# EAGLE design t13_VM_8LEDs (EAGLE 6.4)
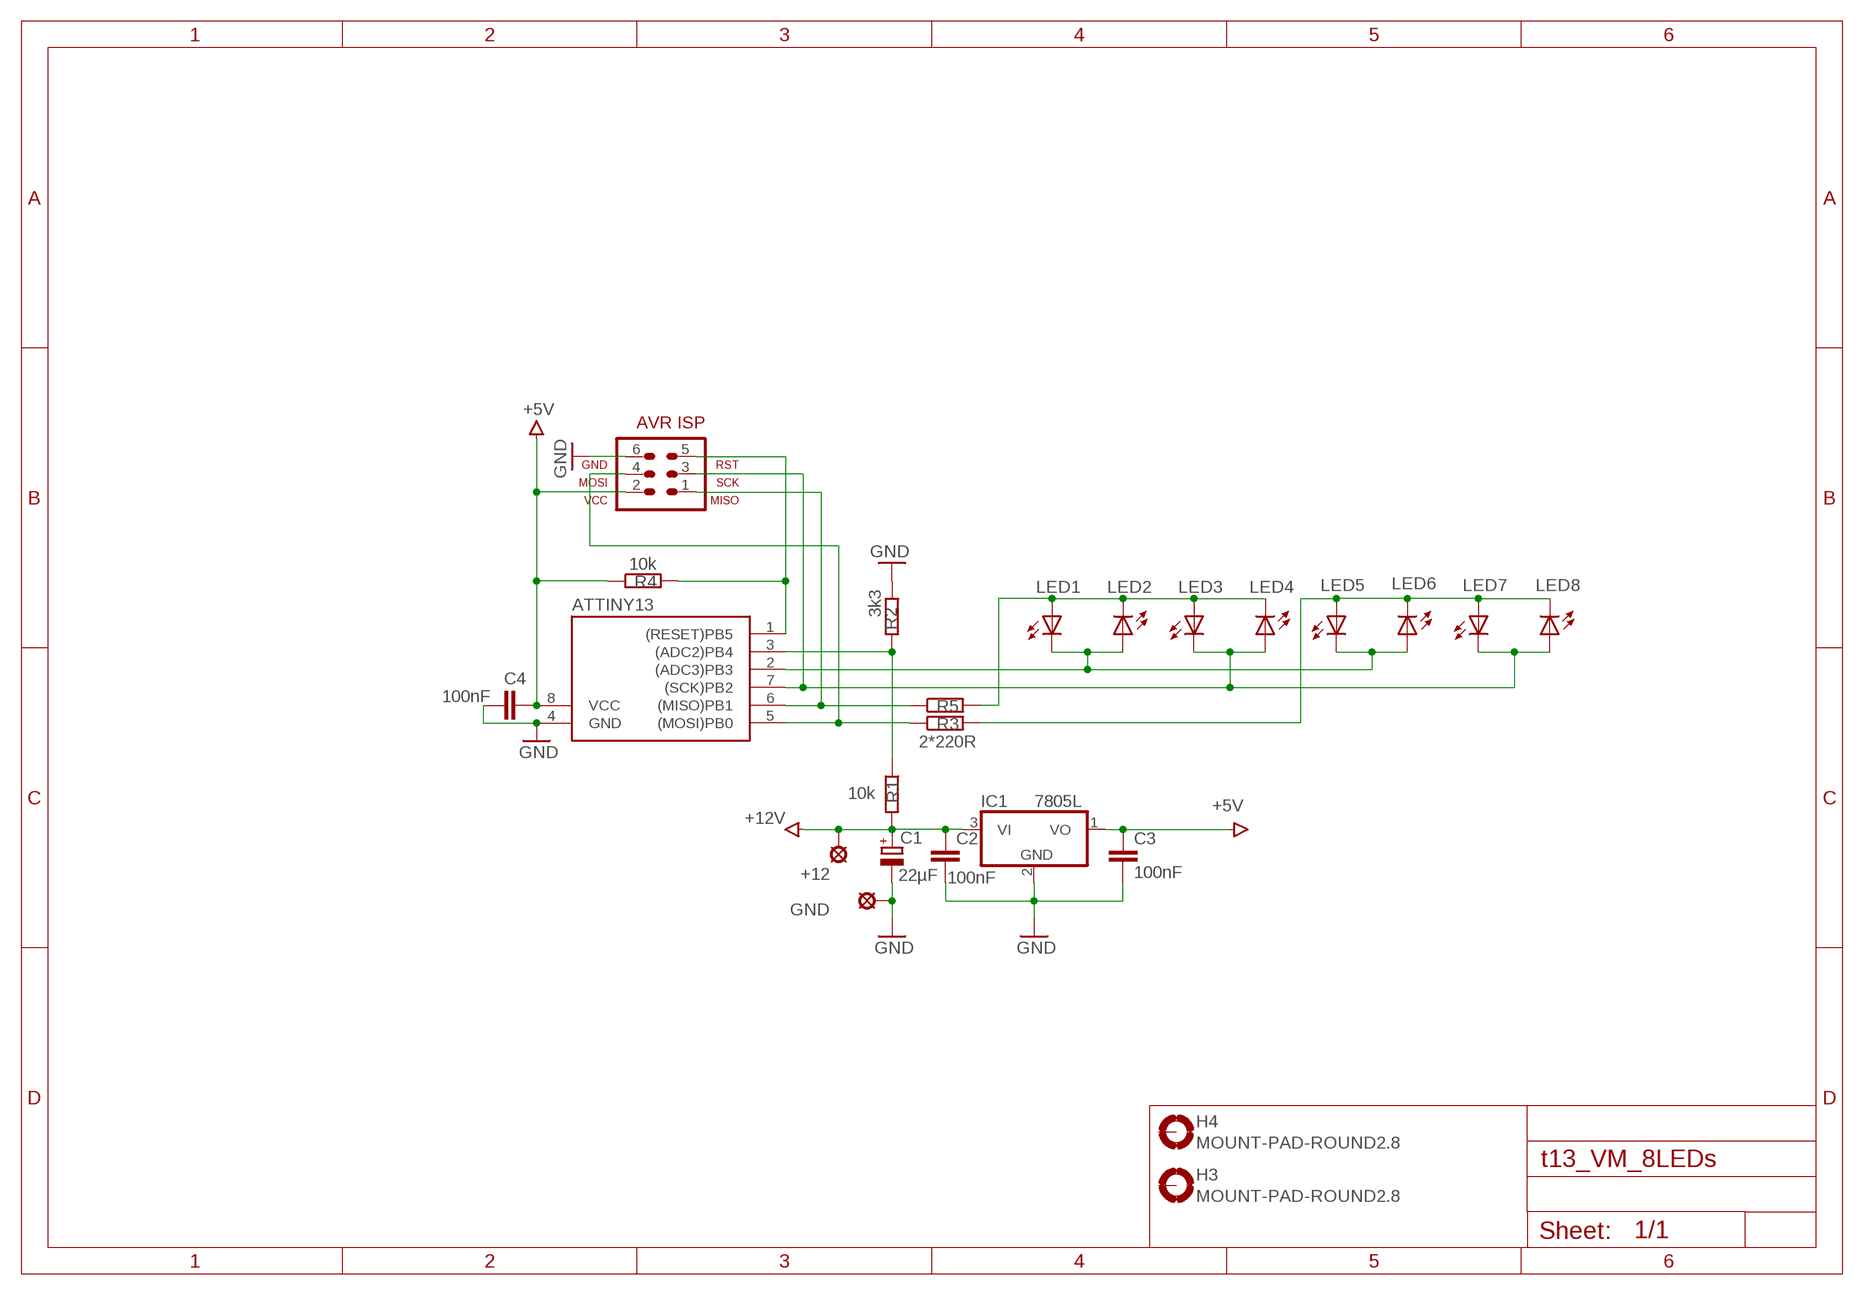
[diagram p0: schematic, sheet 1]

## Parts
+12  LSP10  [LSP10]
ATTINY13  TINY138P3  [DIL08]
C1  22µF  CPOL-EUE2.5-7  [E2,5-7]
C2  100nF  C-EU025-025X050  [C025-025X050]
C3  100nF  C-EU025-025X050  [C025-025X050]
C4  100nF  C-EU025-025X050  [C025-025X050]
GND  GND  LSP10  [LSP10]
H3  MOUNT-PAD-ROUND2.8  [2,8-PAD]
H4  MOUNT-PAD-ROUND2.8  [2,8-PAD]
IC1  7805L  [TO92]
JP1  AVR-ISP-6HORZ  [AVR-ISP-6R]
LED1  LED3MM  [LED3MM]
LED2  LED3MM  [LED3MM]
LED3  LED3MM  [LED3MM]
LED4  LED3MM  [LED3MM]
LED5  LED3MM  [LED3MM]
LED6  LED3MM  [LED3MM]
LED7  LED3MM  [LED3MM]
LED8  LED3MM  [LED3MM]
R1  10k  R-EU_0207/10  [0207/10]
R2  3k3  R-EU_0207/10  [0207/10]
R3  2*220R  R-EU_0207/10  [0207/10]
R4  10k  R-EU_0207/7  [0207/7]
R5  R-EU_0207/10  [0207/10]

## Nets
+5V: ATTINY13.8(VCC) C3.1 C4.2 IC1.1(VO) JP1.2 R4.1
+12V: +12.MP C1.+ C2.1 IC1.3(VI) R1.2
GND: ATTINY13.4(GND) C1.- C2.2 C3.2 C4.1 GND.MP IC1.2(GND) JP1.6 R2.1
N$1: ATTINY13.3((ADC2)PB4) R1.1 R2.2
N$3: LED1.A LED2.K(C) LED3.A LED4.K(C) R5.2
N$4: LED5.A LED6.K(C) LED7.A LED8.K(C) R3.2
N$5: ATTINY13.7((SCK)PB2) JP1.3 LED3.K(C) LED4.A LED7.K(C) LED8.A
N$6: ATTINY13.5((MOSI)PB0) JP1.4 R3.1
N$7: ATTINY13.2((ADC3)PB3) LED1.K(C) LED2.A LED5.K(C) LED6.A
N$9: ATTINY13.1((RESET)PB5) JP1.5 R4.2
N$10: ATTINY13.6((MISO)PB1) JP1.1 R5.1
Unconnected: H3.B2,8(MOUNT) H4.B2,8(MOUNT)

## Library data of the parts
+12 GND = solpad:LSP10: SOLDER PAD
ATTINY13 = avr-5-4.16:TINY13*
C1 = rcl:CPOL-EU: POLARIZED CAPACITOR, European symbol
C2-C4 = rcl:C-EU: CAPACITOR, European symbol
H3 H4 = holes:MOUNT-PAD-ROUND: MOUNTING PAD, round
IC1 = linear:78*: Positive VOLTAGE REGULATOR Source: http://cache.national.com/ds/LM/LM78L05.pdf http://www.fairchildsemi.com/ds/LM/LM7805.pdf
JP1 = avr-7:AVR-ISP-6: AVR ISP-6 Serial Programming Header
LED1-LED8 = led:LED: LED
R1-R5 = rcl:R-EU_: RESISTOR, European symbol

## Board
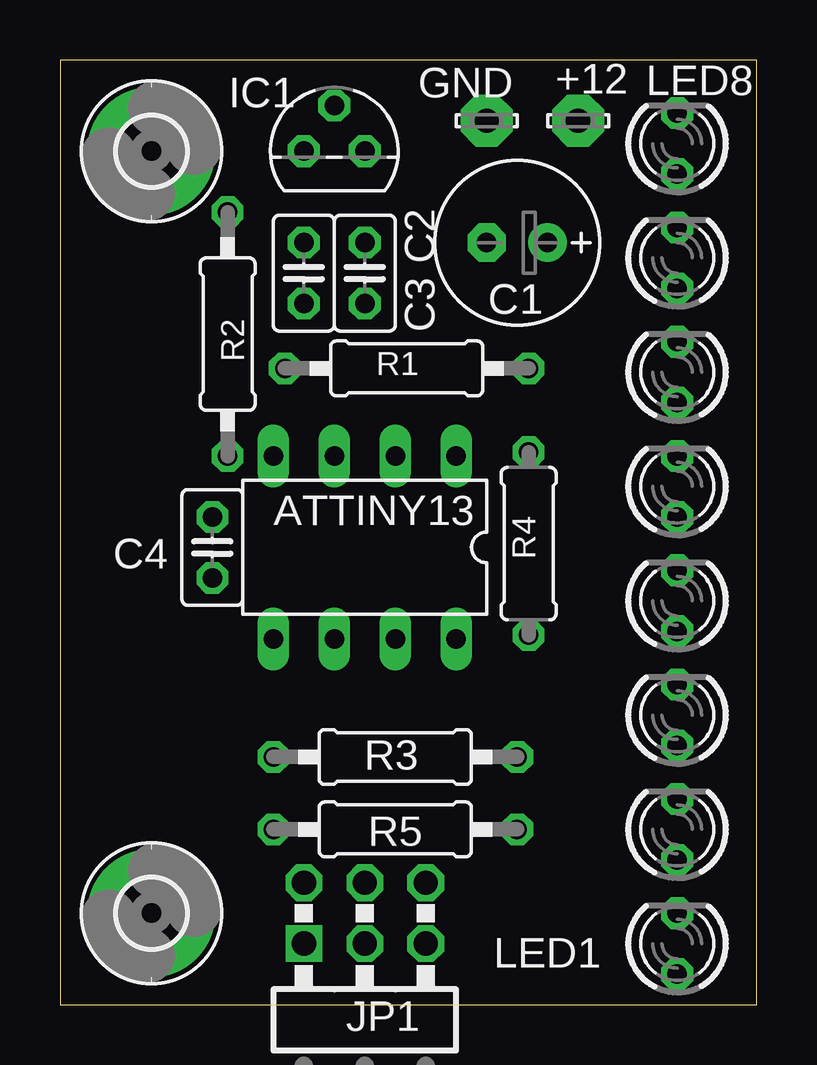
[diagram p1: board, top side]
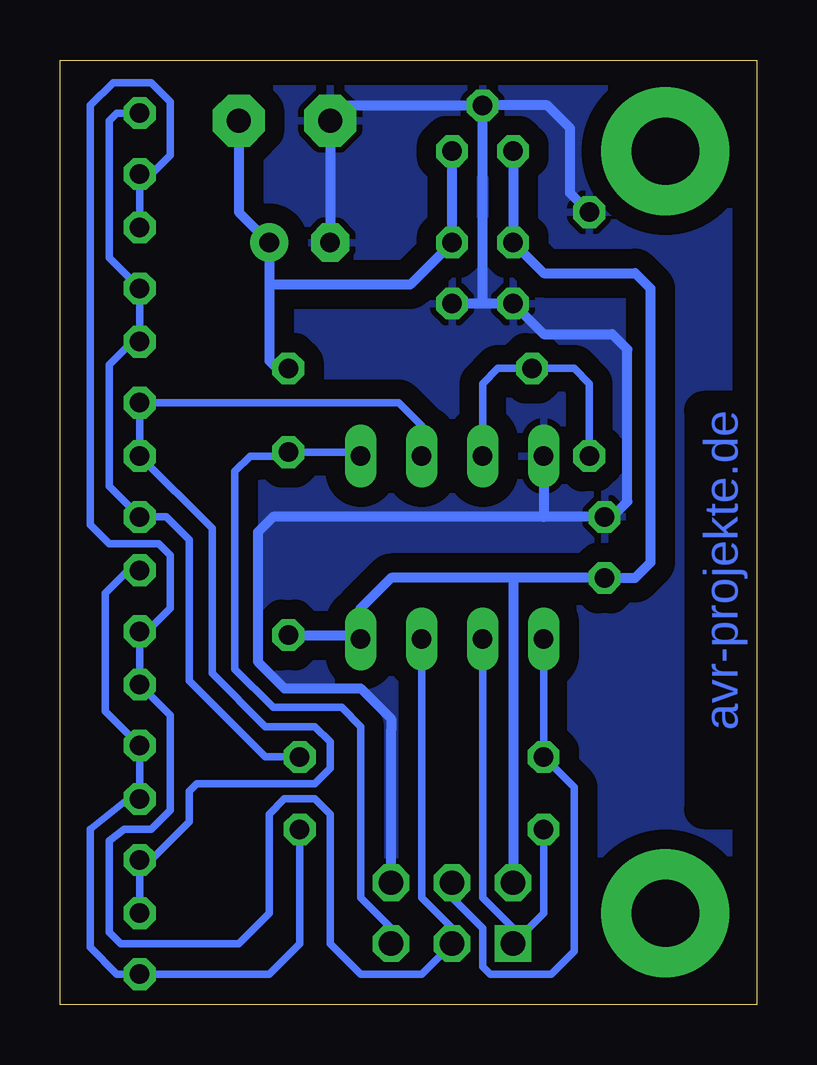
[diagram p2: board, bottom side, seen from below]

Size 29.04 x 39.36 mm. Coordinates in mm from the lower left corner, seen from the top.
Outline: 0,0 29.04,0 29.04,39.36 0,39.36 0,0
Copper layers (1*16): Top 0.035mm / dielectric 1.5mm / Bottom 0.035mm
Design rules "default": minimum track width 10mil, minimum drill 24mil, track to track 8mil, track to pad 8mil, pad to pad 8mil, via to via 8mil, smd to smd 8mil, copper to edge 40mil, drill to drill 8mil, minimum pad ring 10mil, minimum via ring 8mil, stop-mask expansion 4mil, vias tented up to drill 0mil, thermal gap 10mil

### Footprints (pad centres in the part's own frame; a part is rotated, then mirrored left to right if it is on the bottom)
LSP10 = drill 1.016 pad 2.159 octagon: MP 0,0
DIL08 = drill 0.813 long: 1 -3.81,-3.81; 2 -1.27,-3.81; 3 1.27,-3.81; 4 3.81,-3.81; 5 3.81,3.81; 6 1.27,3.81; 7 -1.27,3.81; 8 -3.81,3.81
E2,5-7 = drill 0.813 pad 1.6: + -1.27,0 | drill 0.813 pad 1.6 octagon: - 1.27,0
C025-025X050 = drill 0.813 octagon: 1 -1.27,0; 2 1.27,0
2,8-PAD = drill 2.8 pad 5.334: B2,8 0,0
TO92 = drill 0.813 octagon: 1 -1.27,0; 2 0,1.905; 3 1.27,0
AVR-ISP-6R = drill 1.016 square: 1 -2.54,-1.27 | drill 1.016 octagon: 2 -2.54,1.27; 3 0,-1.27; 4 0,1.27; 5 2.54,-1.27; 6 2.54,1.27
LED3MM = drill 0.813 octagon: A -1.27,0; K 1.27,0
0207/10 = drill 0.813 octagon: 1 -5.08,0; 2 5.08,0
0207/7 = drill 0.813 octagon: 1 -3.81,0; 2 3.81,0

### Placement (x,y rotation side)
+12  21.59,36.83 0 top
ATTINY13  12.7,19.05 180 top
C1  19.05,31.75 180 top
C2  12.7,30.48 270 top
C3  10.16,30.48 270 top
C4  6.35,19.05 270 top
GND  17.78,36.83 0 top
H3  3.81,35.56 0 top
H4  3.81,3.81 0 top
IC1  11.43,35.56 0 top
JP1  12.7,3.81 0 top
LED1  25.72,2.54 90 top
LED2  25.72,7.3 90 top
LED3  25.72,12.06 90 top
LED4  25.72,16.83 90 top
LED5  25.72,21.59 90 top
LED6  25.72,26.35 90 top
LED7  25.72,31.11 90 top
LED8  25.72,35.88 90 top
R1  14.45,26.51 0 top
R2  6.99,27.94 270 top
R3  13.97,10.32 0 top
R4  19.53,19.21 90 top
R5  13.97,7.3 0 top

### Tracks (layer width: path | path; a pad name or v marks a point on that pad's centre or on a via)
+5V
  Bottom 0.305: 16.51,16.51 ATTINY13.8 16.51,15.4
  Bottom 0.406: IC1.1 C3.1 8.89,30.48 5.08,30.48 4.45,29.84 4.45,18.41 5.08,17.78 C4.2 10.16,17.78 | 10.16,17.78 JP1.2 | 10.16,17.78 15.24,17.78 16.51,16.51 | R4.1 16.51,15.4
+12V
  Bottom 0.305: R1.2 20,26.51
  Bottom 0.406: +12.MP 21.59,33.02 C1.+ 20.32,30 | 20.32,30 20.32,26.83 20,26.51 | IC1.3 C2.1 14.45,30 15.72,30 16.51,30 20.32,30
GND
  Bottom 0.305: GND.MP 17.14,37.47 | C4.1 6.03,20.32
  Bottom 0.406: GND.MP C1.- | 17.14,37.47 IC1.2 | 11.43,29.21 C3.2 8.89,27.94 6.03,27.94 5.4,27.3 5.4,20.95 6.03,20.32 | 11.43,29.21 C2.2 | 11.43,29.21 IC1.2 | R2.1 7.78,33.81 7.78,36.51 8.73,37.47 IC1.2 | C4.1 8.89,20.32 | 8.89,20.32 20.16,20.32 20.8,19.68 20.8,14.29 19.68,13.18 16.51,13.18 15.24,11.91 15.24,11.43 JP1.6 | ATTINY13.4 8.89,20.32
  pour Bottom (isolate 0.813): 0,39.37 29.21,39.37 29.21,0 0,0
N$1
  Bottom 0.305: ATTINY13.3 11.43,25.88 10.79,26.51 R1.1 7.62,26.51 6.99,25.88 R2.2
N$3
  Bottom 0.305: R5.2 19.05,2.54 20.32,1.27 LED1.A 26.67,1.27 27.78,2.38 27.78,7.3 26.19,8.57 LED2.K LED3.A 27.15,12.22 27.15,17.14 26.19,18.1 LED4.K
N$4
  Bottom 0.305: LED8.K 26.67,37.15 26.99,36.83 26.99,31.11 LED7.A LED6.K 26.04,27.62 26.99,26.67 26.99,21.59 LED5.A 24.61,20.32 23.65,19.37 23.65,13.49 20.48,10.32 R3.2
N$5
  Bottom 0.305: LED7.K LED8.A 25.24,34.61 24.45,35.4 24.45,37.62 25.24,38.42 26.83,38.42 27.78,37.47 27.78,20 26.99,19.21 24.92,19.21 24.45,18.73 24.45,16.51 25.4,15.56 LED4.A LED3.K 24.45,12.06 24.45,8.1 25.24,7.3 26.35,7.3 26.99,6.83 26.99,3.02 26.51,2.54 21.59,2.54 20.32,3.81 20.32,7.94 19.68,8.57 18.41,8.57 17.78,7.94 17.78,2.54 16.51,1.27 13.97,1.27 JP1.3 12.7,3.17 13.97,4.45 ATTINY13.7
N$6
  Bottom 0.305: JP1.4 12.7,4.45 11.43,3.17 11.43,1.59 11.11,1.27 8.57,1.27 7.62,2.22 7.62,9.05 R3.1 ATTINY13.5
N$7
  Bottom 0.305: ATTINY13.2 13.97,24.13 14.92,25.08 LED6.A LED5.K | LED1.K LED2.A | 25.56,22.7 LED5.K | LED5.K 22.7,19.84 22.7,13.81 20.48,11.59 18.41,11.59 17.78,10.95 17.78,9.84 18.41,9.21 23.34,9.21 23.65,8.89 23.65,7.62 25.24,6.03 LED2.A | 25.56,6.03 LED2.A
N$9
  Bottom 0.305: JP1.5 15.24,3.17 16.51,4.45 16.51,11.59 17.3,12.38 20.16,12.38 21.75,13.97 21.75,22.23 21.11,22.86 19.53,22.86 R4.2 16.51,23.02 ATTINY13.1
N$10
  Bottom 0.305: ATTINY13.6 11.43,4.45 10.16,3.17 JP1.1 8.89,3.81 R5.1

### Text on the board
Bottom: avr-projekte.de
